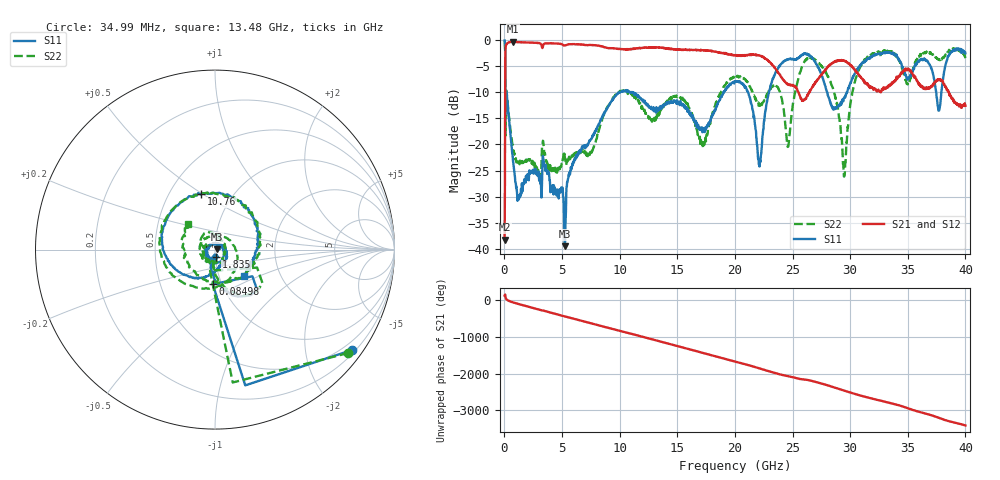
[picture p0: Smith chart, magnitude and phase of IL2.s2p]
!Agilent Technologies,N5230A,US43500312,A.07.50.67
!Agilent N5230A: A.07.50.67
!Date: Wednesday, December 30, 2015 19:51:38
!Correction: S11(Full 2 Port(1,2))
!S21(Full 2 Port(1,2))
!S12(Full 2 Port(1,2))
!S22(Full 2 Port(1,2))
!S2P File: Measurements: S11, S21, S12, S22:
# Hz S  dB  R 50
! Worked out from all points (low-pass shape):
!   1601 points, 10 MHz to 40 GHz, reference 50 ohm
!   highest |S21| = -0.33 dB at 709.8 MHz (marker M1); lowest = -38.2 dB at 10 MHz (marker M2)
!   |S21| within 3 dB of the highest: 79.68 MHz to 22.51 GHz (22.43 GHz wide, 199 % of centre)
!   lowest |S11| = -39.5 dB at 5.234 GHz (marker M3), VSWR 1.02, Z = 51.1 + j0.138 ohm
!   |S11| at or under -10 dB: 171 MHz to 10.06 GHz (9.888 GHz wide, 193 % of centre); 11.06 GHz to 19.02 GHz (7.96 GHz wide, 52.9 % of centre); 21.13 GHz to 22.95 GHz (1.821 GHz wide, 8.26 % of centre)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
!   |S22| runs from -26.6 to -0.2 dB; largest |S21 - S12| = 0.025
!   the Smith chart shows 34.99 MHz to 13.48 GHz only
!   S11 on the Smith chart (normalised r, x): 34.99 MHz: 0.28, -3.04; 84.98 MHz: 0.91, -0.36; 1.835 GHz: 1.01, -0.09; 10.76 GHz: 0.72, +0.49; 13.48 GHz: 1.31, -0.41
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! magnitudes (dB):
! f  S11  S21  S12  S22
! 10 MHz  -0.1  -38.2  -38.2  -0.2
! 34.99 MHz  -0.5  -29.3  -29.3  -0.5
! 84.98 MHz  -14.3  -1.8  -1.8  -18.4
! 259.9 MHz  -12.0  -0.6  -0.6  -11.8
! 709.8 MHz  -22.2  -0.3  -0.3  -20.1
! 1.835 GHz  -27.3  -0.5  -0.5  -23.3
! 5.234 GHz  -39.5  -1.1  -1.0  -22.3
! 6.683 GHz  -20.8  -0.9  -0.9  -21.4
! 10.76 GHz  -10.0  -1.8  -1.8  -10.0
! 13.36 GHz  -13.1  -1.5  -1.5  -13.8
! 13.48 GHz  -13.3  -1.5  -1.5  -13.8
! 17.23 GHz  -17.2  -2.0  -1.9  -20.7
! 20 GHz  -8.0  -2.9  -2.9  -7.1
! 22.13 GHz  -24.2  -3.0  -3.0  -12.2
! 23.68 GHz  -5.7  -6.1  -6.0  -9.0
! 24.63 GHz  -3.8  -8.6  -8.6  -20.4
! 26.68 GHz  -3.4  -9.2  -9.3  -3.6
! 29.5 GHz  -11.0  -4.1  -4.0  -26.0
! 30.75 GHz  -5.3  -6.7  -6.7  -5.8
! 33.35 GHz  -2.4  -8.8  -8.8  -2.3
! 37.7 GHz  -13.6  -7.6  -7.5  -3.8
! 40 GHz  -2.6  -12.6  -12.7  -3.5
